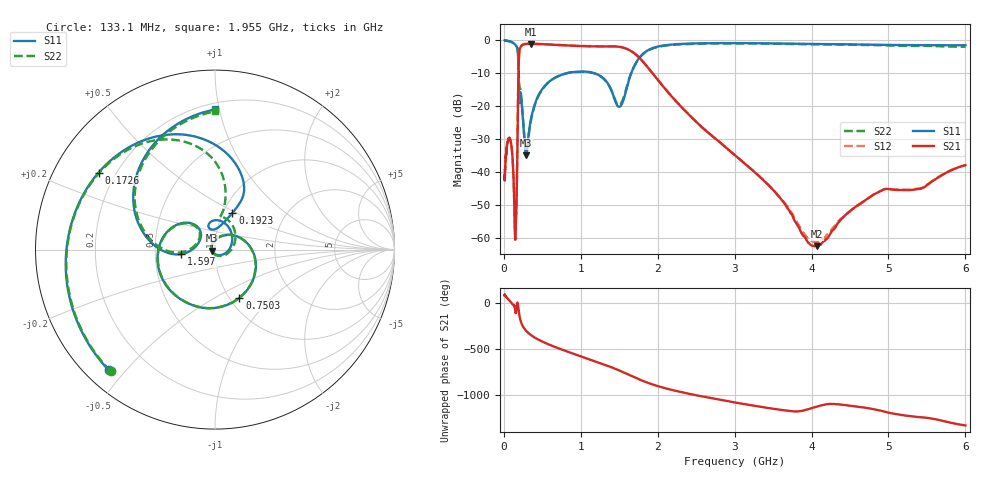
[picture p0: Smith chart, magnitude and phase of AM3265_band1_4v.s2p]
!Agilent Technologies,E8364B,MY43040894,A.07.50.67
!Agilent E8364B: A.07.50.67
!Date: Friday, May 09, 2025 07:15:18
!Correction: S11(Full 2 Port(1,2))
!S21(Full 2 Port(1,2))
!S12(Full 2 Port(1,2))
!S22(Full 2 Port(1,2))
!S2P File: Measurements: S11, S21, S12, S22:Log Frequency Sweep
# Hz S  dB  R 50
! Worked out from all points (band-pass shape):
!   3201 points, 10 MHz to 6 GHz, reference 50 ohm
!   highest |S21| = -1.03 dB at 351 MHz (marker M1); lowest = -62.4 dB at 4.071 GHz (marker M2)
!   |S21| within 3 dB of the highest: 198.8 MHz to 1.703 GHz (1.505 GHz wide, 158 % of centre)
!   lowest |S11| = -34.8 dB at 290.3 MHz (marker M3), VSWR 1.04, Z = 48.3 - j0.592 ohm
!   |S11| at or under -10 dB: 190 MHz to 807.4 MHz (617.4 MHz wide, 124 % of centre); 1.186 GHz to 1.655 GHz (469.1 MHz wide, 33 % of centre)
!   |S22| runs from -33.9 to 0.0 dB; largest |S21 - S12| = 0.0043
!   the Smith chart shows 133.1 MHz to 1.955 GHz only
!   S11 on the Smith chart (normalised r, x): 133.1 MHz: 0.07, -0.45; 172.6 MHz: 0.14, +0.30; 192.3 MHz: 1.11, +0.48; 750.3 MHz: 1.11, -0.66; 1.597 GHz: 0.68, -0.04; 1.955 GHz: 0.24, +0.97
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1e7  -0.02 -8.2  -41.93 82.2  -42.37 89.5  -0.07 -8.3
2.908064e7  -0.06 -23.7  -34.40 68.2  -34.17 66.7  -0.06 -23.8
8.439949e7  -0.31 -73.2  -30.12 16.0  -30.07 16.5  -0.34 -73.3
1.331322e8  -0.96 -131.5  -47.56 -30.2  -47.39 -31.0  -0.98 -130.6
1.492e8  -1.32 -157.7  -59.83 -90.3  -58.26 23.5  -1.33 -156.0
1.726416e8  -2.18 146.6  -39.03 -6.7  -39.21 -8.0  -2.11 152.2
1.92321e8  -12.88 64.6  -7.64 -70.4  -7.60 -70.4  -8.95 80.9
2.129627e8  -15.74 90.8  -2.20 -178.3  -2.17 -178.2  -14.68 72.7
2.44949e8  -22.95 -7.6  -1.30 111.4  -1.27 111.4  -22.29 -13.2
2.903155e8  -34.84 -160.2  -1.07 57.8  -1.03 57.7  -33.87 -154.3
3.510319e8  -24.05 79.3  -1.03 12.9  -0.99 12.9  -24.42 84.0
7.123273e8  -10.78 -52.5  -1.40 -132.0  -1.36 -132.0  -10.79 -53.0
7.503296e8  -10.43 -63.1  -1.44 -143.9  -1.41 -143.9  -10.44 -63.6
1.18121e9  -9.96 -178.2  -1.79 89.8  -1.77 89.8  -10.03 -179.1
1.597428e9  -14.45 -172.2  -2.55 -47.2  -2.53 -47.2  -14.09 -175.2
1.954819e9  -2.15 89.9  -10.60 -168.9  -10.58 -168.9  -2.27 89.8
2.067357e9  -1.55 62.8  -13.85 163.3  -13.81 163.2  -1.68 63.1
2.455151e9  -0.91 -11.0  -23.66 87.6  -23.65 87.8  -1.05 -10.4
2.96862e9  -0.79 -90.1  -34.10 7.0  -34.11 6.8  -0.90 -90.3
4.071232e9  -1.07 121.2  -62.42 -42.9  -61.15 -42.3  -1.18 118.8
5.002045e9  -1.35 4.3  -45.08 -108.6  -45.10 -108.5  -1.53 4.8
6e9  -1.44 -115.1  -37.85 112.8  -37.83 112.1  -1.95 -110.9
